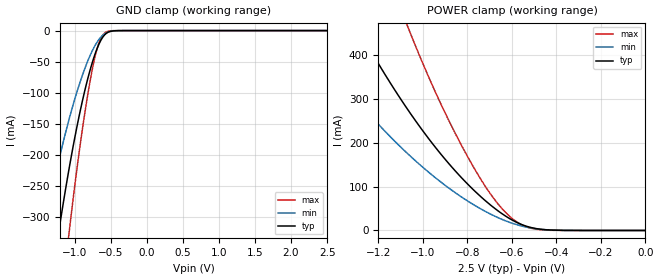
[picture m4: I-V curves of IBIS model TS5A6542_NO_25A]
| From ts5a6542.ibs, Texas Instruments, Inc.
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[Model]   TS5A6542_NO_25A
Model_type  Terminator
| variable   typ   min   max
C_comp   37.66pF   34.04pF   41.88pF
| C_tri-state   37.66pF   34.04pF   41.88pF
[Temperature Range]   40   100   -40
| Ambient temperature   25   85   -40
[Voltage range]   2.5   2.25   2.75
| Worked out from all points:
|   GND clamp passes 1 mA (typ) near -0.49 V on its own axis
|   POWER clamp passes 1 mA (typ) near -0.43 V on its own axis
[GND Clamp]
| TS5A6542_NO_25A
|   Voltage   I(typ)   I(min)   I(max)
-2.5V     -1.624A    -1.127A    -2.268A
-1.43V    -494.9mA   -324.2mA   -729.2mA
-1.225V   -327.8mA   -212.3mA   -484.1mA
-1.2V     -309.1mA   -199.8mA   -456.2mA
-1.085V   -228mA     -146.5mA   -334.2mA
-1.065V   -214.9mA   -137.9mA   -314.2mA
-920mV    -128.3mA   -81.59mA   -181.7mA
-770mV    -57.49mA   -36.29mA   -71.74mA
-670mV    -23.93mA   -15.58mA   -22.5mA
-565mV    -4.897mA   -3.969mA   -2.497mA
-385mV    -56.34uA   -94.65uA   -5.746uA
2.5V      1.521nA    17.37uA    48.44pA
[POWER Clamp]
| TS5A6542_NO_25A
|   Voltage   I(typ)   I(min)   I(max)
-2.5V     1.969A     1.329A     3.101A
-1.545V   711.4mA    458.3mA    1.19A
-1.28V    449mA      286.3mA    759mA
-1.075V   279.9mA    177.7mA    471.9mA
-1.055V   265.1mA    168.2mA    446.5mA
-915mV    170.9mA    108.4mA    282.9mA
-780mV    95.85mA    60.96mA    150.5mA
-690mV    55.28mA    35.66mA    78.42mA
-600mV    24.01mA    16.63mA    27.64mA
-540mV    10.44mA    8.132mA    9.271mA
-470mV    2.74mA     2.625mA    1.548mA
-31.15fV  1.521nA    12.57nA    64.13pA
